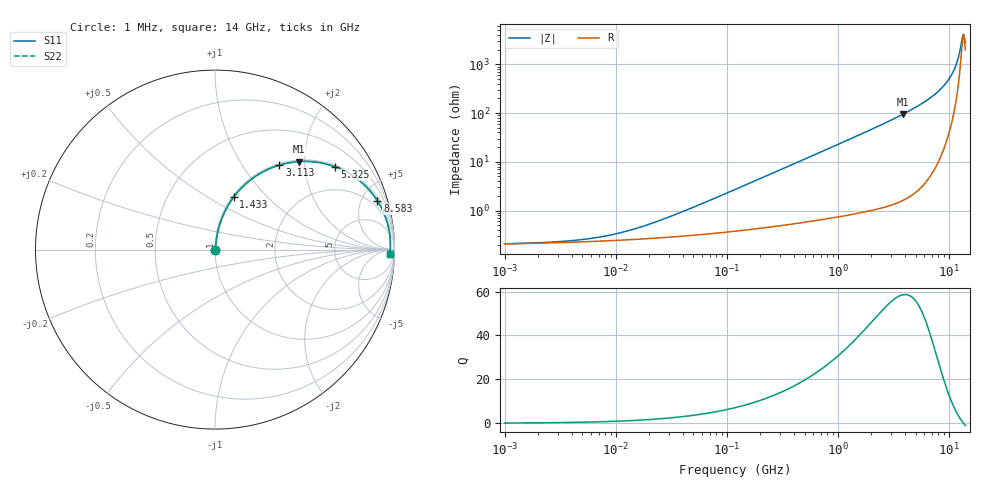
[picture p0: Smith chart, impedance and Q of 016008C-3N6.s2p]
# MHz S MA R 50
!Freq  MagS11  AngS11  MagS21  AngS21  MagS12  AngS12  MagS22  AngS22
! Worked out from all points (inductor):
!   801 points, 1 MHz to 14 GHz, reference 50 ohm
!   read as one part in series: L = 3.6 nH near 39.94 MHz
!   highest Q = 58.5 at 3.813 GHz (marker M1), where L = 3.92 nH
!   self-resonance near 13.35 GHz
!   S11 on the Smith chart (normalised r, x): 1 MHz: 1.00, +0.00; 1.433 GHz: 1.02, +0.66; 3.113 GHz: 1.03, +1.49; 5.325 GHz: 1.05, +2.86; 8.583 GHz: 1.29, +6.54; 14 GHz: 40, -39
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1  0.00208 6.2  0.9979 -0.0  0.9979 -0.0  0.00208 6.2
2.536574  0.002244 14.8  0.9978 -0.0  0.9978 -0.0  0.002244 14.8
4.948533  0.002537 26.1  0.9977 -0.1  0.9977 -0.1  0.002537 26.1
10.87757  0.003476 44.8  0.9975 -0.1  0.9975 -0.1  0.003476 44.8
24.19749  0.006107 63.0  0.9972 -0.3  0.9972 -0.3  0.006107 63.0
119.742  0.02724 80.5  0.9959 -1.5  0.9959 -1.5  0.02724 80.5
289.5766  0.06525 82.1  0.9931 -3.7  0.9931 -3.7  0.06525 82.1
585.5183  0.1309 79.9  0.9854 -7.5  0.9854 -7.5  0.1309 79.9
1432.979  0.3093 70.5  0.9429 -18.0  0.9429 -18.0  0.3093 70.5
2049.839  0.4254 63.6  0.8959 -25.2  0.8959 -25.2  0.4254 63.6
2863.085  0.5567 55.1  0.8205 -33.8  0.8205 -33.8  0.5567 55.1
3112.525  0.5919 52.7  0.7955 -36.3  0.7955 -36.3  0.5919 52.7
3812.572  0.6784 46.3  0.7232 -42.7  0.7232 -42.7  0.6784 46.3
5325.159  0.8122 34.6  0.5684 -54.3  0.5684 -54.3  0.8122 34.6
6923.905  0.8965 24.9  0.4206 -63.7  0.4206 -63.7  0.8965 24.9
8582.997  0.9449 16.8  0.2886 -70.7  0.2886 -70.7  0.9449 16.8
9786.969  0.9641 11.8  0.2053 -74.1  0.2053 -74.1  0.9641 11.8
10767.37  0.9729 8.2  0.1445 -75.1  0.1445 -75.1  0.9729 8.2
11845.97  0.9773 4.7  0.08425 -72.1  0.08425 -72.1  0.9773 4.7
13032.63  0.9773 1.2  0.03055 -41.5  0.03055 -41.5  0.9773 1.2
13507.66  0.9762 -0.1  0.02391 5.1  0.02391 5.1  0.9762 -0.1
14000  0.9744 -1.4  0.03551 43.2  0.03551 43.2  0.9744 -1.4
